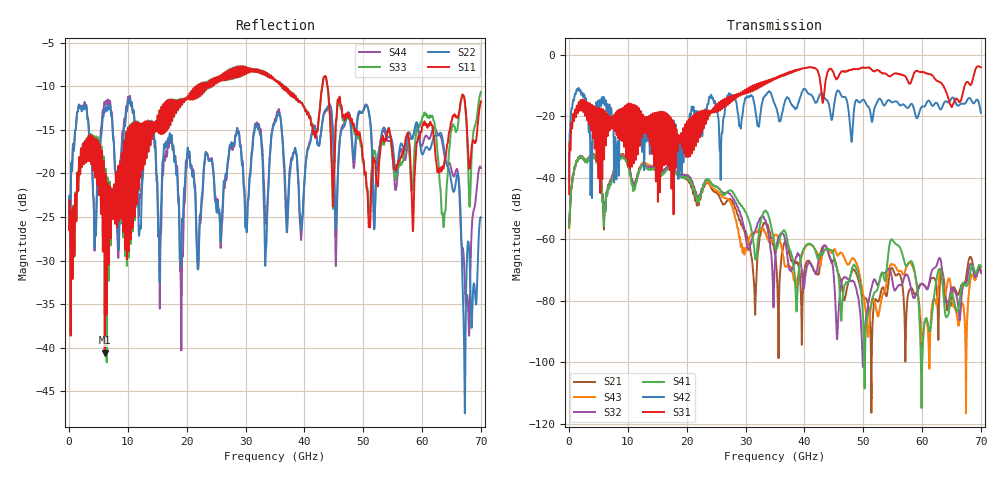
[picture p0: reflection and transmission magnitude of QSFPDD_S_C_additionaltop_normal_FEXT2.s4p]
! AWR Design Environment (8415) Thu Dec 20 12:55:39 2018
! Document = 'CHANNEL TEST'
! nPorts: 4, nXvals: 7001
# HZ S DB R 50
!Freq DBS11 AngS11 DBS12 AngS12 DBS13 AngS13 DBS14 AngS14
!	DBS21 AngS21 DBS22 AngS22 DBS23 AngS23 DBS24 AngS24
!	DBS31 AngS31 DBS32 AngS32 DBS33 AngS33 DBS34 AngS34
!	DBS41 AngS41 DBS42 AngS42 DBS43 AngS43 DBS44 AngS44
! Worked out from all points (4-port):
!   7000 points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, 10 MHz to 70 GHz, reference 50 ohm
!   strongest paths, dB at 10 MHz, 17.51 GHz, 35.01 GHz, 52.51 GHz, 70 GHz:
!     S31: -45.3, -23.9, -7.5, -5.0, -4.0
!     S42: -41.3, -22.5, -16.2, -14.8, -18.8
!     S41: -56.0, -37.0, -62.2, -75.6, -68.9
!     S32: -55.6, -36.5, -67.3, -74.8, -70.9
!     S43: -56.4, -36.3, -58.5, -85.1, -68.9
!     S21: -55.5, -36.7, -64.8, -80.3, -70.3
!   lowest |S11| = -40.5 dB at 6.06 GHz (marker M1), VSWR 1.02, Z = 49.4 + j0.738 ohm
!   |S11| at or under -10 dB: start of sweep to 21.77 GHz; 36.5 GHz to 43.04 GHz (6.538 GHz wide, 16.4 % of centre); 43.94 GHz to end of sweep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
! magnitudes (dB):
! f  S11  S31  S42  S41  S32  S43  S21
! 10 MHz  -26.5  -45.3  -41.3  -56.0  -55.6  -56.4  -55.5
! 1.91 GHz  -19.7  -15.2  -11.4  -32.9  -32.9  -33.0  -32.8
! 6.06 GHz  -40.5  -18.8  -16.4  -49.1  -47.9  -50.0  -50.5
! 9.1 GHz  -20.2  -23.1  -24.0  -33.3  -32.8  -32.5  -32.3
! 27.55 GHz  -8.0  -13.8  -13.0  -44.2  -45.7  -48.5  -47.2
! 31.57 GHz  -8.1  -9.7  -16.6  -65.4  -57.7  -57.8  -80.9
! 70 GHz  -11.8  -4.0  -18.8  -68.9  -70.9  -68.9  -70.3
